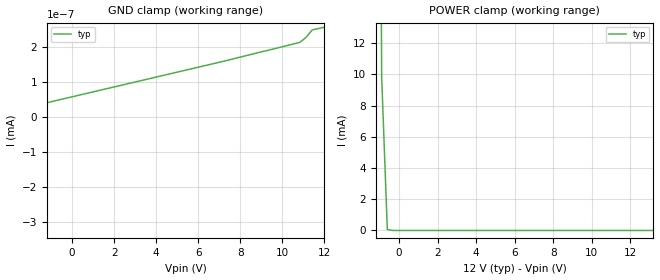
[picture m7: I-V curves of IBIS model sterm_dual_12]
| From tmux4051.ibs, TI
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| sterm_dual_12
[Model]   sterm_dual_12
Model_type   Terminator
|   typ   min   max
C_comp   2.533030e-12   NA   NA
[Voltage Range]   12   NA   NA
[Temperature Range]   27   NA   NA
[Power Clamp Reference]   12   NA   NA
[GND Clamp Reference]   0   NA   NA
[GND Clamp]
|   Voltage   I(typ)   I(min)   I(max)
-17V      -2.321A    NA         NA
-12.61V   -5.738uA   NA         NA
-12.31V   -173.1pA   NA         NA
-12.02V   -138.3pA   NA         NA
-10.85V   -97.64pA   NA         NA
-4.99V    -12.55pA   NA         NA
-4.697V   -84.11pA   NA         NA
-3.525V   81.46pA    NA         NA
-3.232V   12.28pA    NA         NA
10.83V    213.7pA    NA         NA
11.41V    249pA      NA         NA
12V       256.8pA    NA         NA
[POWER Clamp]
|   Voltage   I(typ)   I(min)   I(max)
-5V       1.914A     NA         NA
-1.192V   76.54mA    NA         NA
-899mV    9.847mA    NA         NA
-606.1mV  57.29uA    NA         NA
-313.1mV  12.07nA    NA         NA
24V       -138pA     NA         NA
